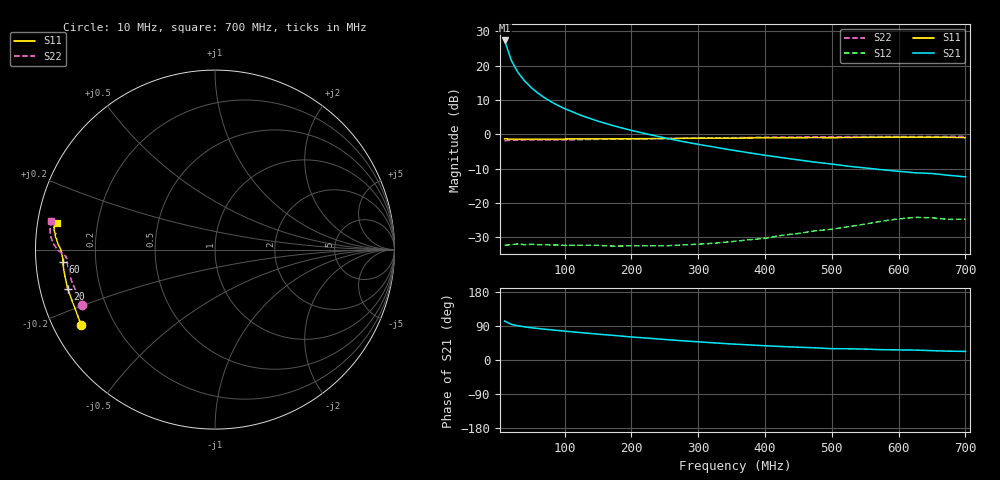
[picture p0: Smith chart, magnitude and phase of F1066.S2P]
! Date: Fri Aug 11 10:32:02 1995
# MHZ  S  MA  R  50.0000
!  POLYFET RF DEVICES
!  F1066 (Each Side)
!  S PARAMETERS
!  VDS=28V, IDQ=800mA
!FREQ  S11MAG S11ANG S21MAG S21ANG S12MAG S12ANG S22MAG S22ANG
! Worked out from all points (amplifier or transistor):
!   34 points, 10 MHz to 700 MHz, reference 50 ohm
!   highest |S21| = 27.4 dB at 10 MHz (marker M1)
!   |S21| within 3 dB of that: start of sweep to 15.17 MHz
!   unconditionally stable (mu >= 1): 160.5 MHz to 573.8 MHz; 683.5 MHz to end of sweep
!   at 60 MHz: K = 0.40, MSG = 22.1 dB, |S12| = -32.2 dB
!   at 300 MHz: K = 1.49, MAG = 10.4 dB, |S12| = -32.1 dB
!   at 700 MHz: K = 1.11, MAG = 4.1 dB, |S12| = -24.7 dB
!   S11 on the Smith chart (normalised r, x): 10 MHz: 0.08, -0.26; 20 MHz: 0.08, -0.13; 60 MHz: 0.08, -0.04; 700 MHz: 0.06, +0.08
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10  0.8563 -150.5  23.31 102.7  0.02411 15.7  0.8038 -157.4
20  0.8493 -165.1  11.95 94.1  0.02448 8.9  0.8194 -168.4
30  0.8493 -170.2  7.953 90.2  0.02518 7.1  0.8205 -172.1
40  0.8502 -172.8  5.971 87.4  0.02454 6.5  0.826 -173.9
50  0.8504 -174.4  4.768 85.2  0.02482 7.8  0.8258 -175.2
60  0.8495 -175.4  3.971 83.1  0.02454 6.5  0.825 -176.0
70  0.8497 -176.3  3.394 81.2  0.02454 7.0  0.8259 -176.4
80  0.8496 -176.7  2.967 79.5  0.02425 9.5  0.8272 -176.7
90  0.8512 -177.3  2.627 77.9  0.02433 8.4  0.8316 -177.0
100  0.852 -177.7  2.362 76.2  0.02394 9.1  0.8292 -177.2
125  0.8547 -178.6  1.875 72.1  0.02409 11.5  0.8352 -177.6
150  0.8554 -178.9  1.55 68.2  0.02401 13.8  0.843 -178.0
175  0.8587 -179.7  1.313 64.6  0.02334 19.4  0.8471 -178.2
200  0.8598 179.9  1.137 60.7  0.02367 21.5  0.8489 -178.4
250  0.8658 178.9  0.8842 54.2  0.02365 28.9  0.8647 -179.2
300  0.8739 178.2  0.7119 48.0  0.02492 38.5  0.8796 180.0
375  0.8823 176.9  0.5382 39.9  0.02884 50.2  0.8967 178.3
475  0.895 174.7  0.3918 32.1  0.03905 60.3  0.9165 175.8
600  0.9057 172.1  0.2881 26.7  0.05832 60.3  0.9272 172.2
625  0.9037 171.6  0.2741 26.1  0.06135 55.4  0.9254 171.5
675  0.9017 170.2  0.252 23.3  0.0573 52.3  0.9301 170.8
700  0.8927 170.3  0.2393 22.6  0.05806 56.0  0.93 170.1
